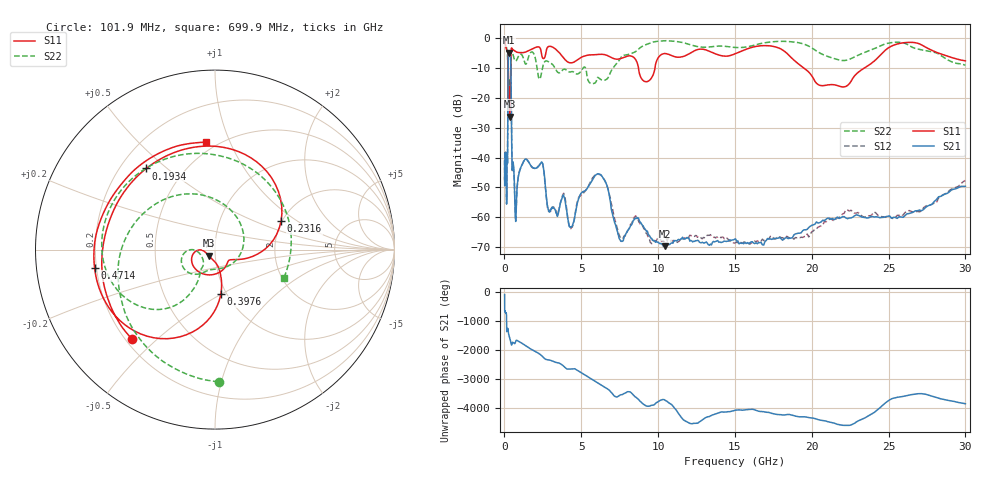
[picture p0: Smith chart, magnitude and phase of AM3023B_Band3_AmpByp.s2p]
# Hz S DB R 50.0
!freq dBS11 angS11 dBS21 angS21 dBS12 angS12 dBS22 angS22
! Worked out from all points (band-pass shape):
!   1601 points, 10 MHz to 30 GHz, reference 50 ohm
!   highest |S21| = -4.86 dB at 282.9 MHz (marker M1); lowest = -69.6 dB at 10.44 GHz (marker M2)
!   |S21| within 3 dB of the highest: 240.2 MHz to 406 MHz (165.8 MHz wide, 51.3 % of centre)
!   lowest |S11| = -26.3 dB at 352.6 MHz (marker M3), VSWR 1.10, Z = 46.5 - j3.09 ohm
!   |S11| at or under -10 dB: 235.8 MHz to 404.2 MHz (168.4 MHz wide, 52.6 % of centre); 8.723 GHz to 9.797 GHz (1.074 GHz wide, 11.6 % of centre); 19.48 GHz to 23.43 GHz (3.953 GHz wide, 18.4 % of centre)
!   |S22| runs from -21.6 to -0.9 dB; largest |S21 - S12| = 0.015
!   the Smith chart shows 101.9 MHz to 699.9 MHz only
!   S11 on the Smith chart (normalised r, x): 101.9 MHz: 0.22, -0.42; 193.4 MHz: 0.31, +0.43; 231.6 MHz: 1.98, +0.75; 397.6 MHz: 0.94, -0.49; 471.4 MHz: 0.19, -0.07; 699.9 MHz: 0.44, +0.82
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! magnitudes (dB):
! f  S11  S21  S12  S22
! 10 MHz  -0.8  -41.4  -40.9  -1.3
! 38.04 MHz  -1.5  -40.3  -39.9  -1.5
! 101.9 MHz  -3.3  -41.3  -40.4  -2.6
! 144.7 MHz  -3.9  -54.1  -53.0  -3.6
! 193.4 MHz  -4.5  -42.0  -41.8  -5.7
! 231.6 MHz  -7.9  -11.8  -11.7  -13.8
! 282.9 MHz  -17.2  -4.9  -4.8  -14.6
! 352.6 MHz  -26.3  -5.0  -4.9  -21.2
! 397.6 MHz  -12.1  -6.6  -6.5  -14.0
! 471.4 MHz  -3.4  -34.8  -34.5  -4.0
! 547.7 MHz  -3.9  -41.5  -41.6  -5.4
! 699.9 MHz  -4.4  -59.0  -58.3  -7.6
! 1.076 GHz  -4.9  -43.1  -43.1  -5.4
! 2.084 GHz  -3.1  -43.4  -43.4  -8.8
! 4.326 GHz  -8.3  -63.2  -63.8  -11.3
! 6.202 GHz  -5.5  -45.6  -45.7  -13.6
! 7.926 GHz  -6.2  -65.3  -65.5  -5.7
! 9.256 GHz  -14.6  -64.7  -65.4  -2.1
! 10.44 GHz  -5.2  -69.6  -67.8  -0.9
! 19.12 GHz  -8.6  -65.3  -66.7  -1.6
! 21.45 GHz  -15.7  -60.8  -61.2  -6.9
! 30 GHz  -7.6  -49.6  -47.6  -9.1
